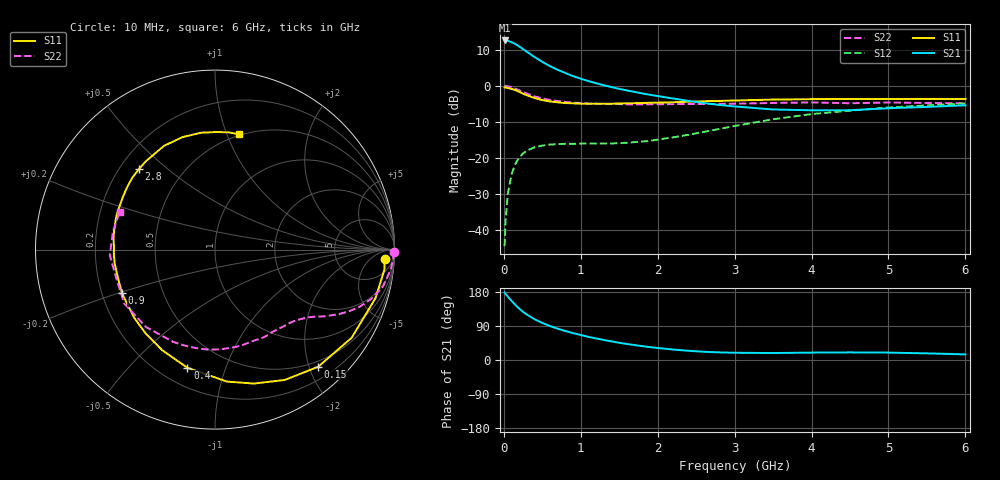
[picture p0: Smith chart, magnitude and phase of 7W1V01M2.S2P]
! Infineon Technologies  Discrete & RF Semiconductors
! BFS17W
! Si NPN RF Bipolar Junction Transistor in SOT323
! VCE = 1 V  IC = 1.2 mA
! Common Emitter S-Parameters:  August  1999
# GHz  S  MA  R  50
!  f  S11  S21  S12  S22
! GHz  MAG  ANG  MAG  ANG  MAG  ANG  MAG  ANG
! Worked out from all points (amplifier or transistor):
!   36 points, 10 MHz to 6 GHz, reference 50 ohm
!   highest |S21| = 12.6 dB at 10 MHz (marker M1)
!   |S21| within 3 dB of that: start of sweep to 289 MHz
!   unconditionally stable (mu >= 1): 903.2 MHz to end of sweep
!   at 250 MHz: K = 0.30, MSG = 14.5 dB, |S12| = -18.8 dB
!   at 1.4 GHz: K = 1.38, MAG = 4.2 dB, |S12| = -16.0 dB
!   at 6 GHz: K = 1.13, MAG = -2.5 dB, |S12| = -4.9 dB
!   S11 on the Smith chart (normalised r, x): 10 MHz: 18, -18; 150 MHz: 0.40, -2.15; 400 MHz: 0.31, -0.75; 900 MHz: 0.28, -0.20; 2.8 GHz: 0.28, +0.40; 6 GHz: 0.49, +1.11
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0.01  0.947 -3.2  4.273 178.3  0.0059 87.0  0.9991 -0.8
0.02  0.9503 -6.9  4.258 175.2  0.0121 87.0  0.9948 -2.6
0.05  0.934 -16.9  4.229 167.6  0.0308 80.4  0.9855 -6.5
0.1  0.9061 -32.8  4.04 156.2  0.0589 71.2  0.9573 -12.5
0.15  0.8698 -48.6  3.812 145.0  0.0823 62.1  0.9119 -17.6
0.2  0.8239 -61.8  3.528 135.5  0.1007 55.5  0.8655 -21.7
0.25  0.7772 -73.8  3.237 127.1  0.115 49.3  0.8192 -24.9
0.3  0.7384 -84.8  2.968 119.8  0.126 44.9  0.7787 -27.5
0.4  0.6762 -103.1  2.511 107.4  0.1401 37.6  0.7139 -31.4
0.5  0.6331 -117.7  2.156 97.8  0.1477 33.0  0.6682 -34.0
0.6  0.6065 -129.4  1.877 89.6  0.1525 29.9  0.6364 -36.5
0.7  0.5896 -139.4  1.669 82.6  0.1549 28.1  0.6149 -39.0
0.9  0.5715 -155.1  1.363 70.9  0.1564 26.5  0.584 -44.2
1.1  0.5625 -167.5  1.165 61.0  0.1574 26.9  0.5689 -49.9
1.6  0.5717 169.9  0.861 42.2  0.1616 33.7  0.5523 -66.0
2.2  0.5909 150.4  0.666 27.6  0.1924 45.4  0.5565 -86.7
2.8  0.617 133.4  0.542 20.1  0.2514 51.0  0.5612 -108.0
3.5  0.6441 116.2  0.469 18.4  0.343 49.0  0.5779 -131.7
4  0.6524 106.1  0.457 19.5  0.4049 43.9  0.5882 -149.3
4.5  0.6558 96.8  0.458 20.1  0.451 38.0  0.5726 -164.5
5.5  0.6579 83.3  0.509 17.5  0.5346 27.0  0.5775 169.8
6  0.6561 78.1  0.537 14.8  0.5681 21.7  0.5711 158.6
